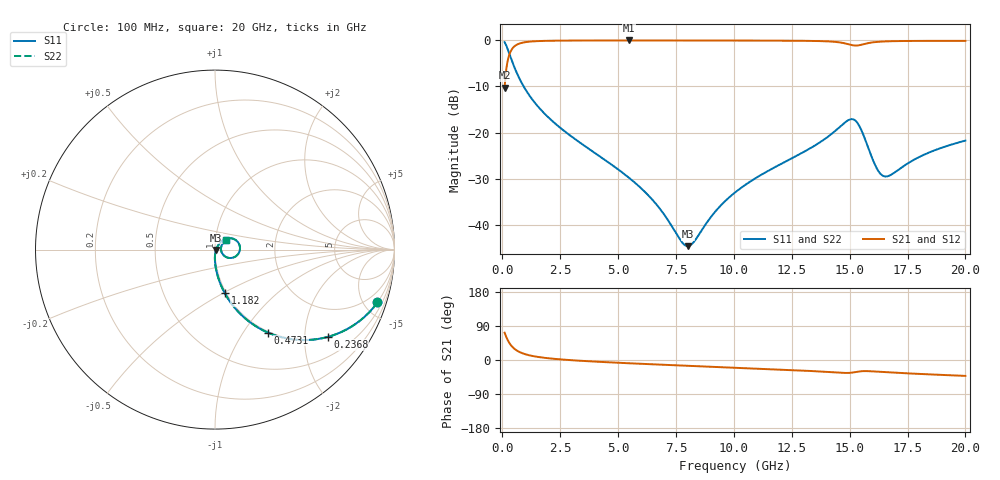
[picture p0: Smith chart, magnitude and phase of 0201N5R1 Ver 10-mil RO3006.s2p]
# GHz S MA R 50
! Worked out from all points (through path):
!   1601 points, 100 MHz to 20 GHz, reference 50 ohm
!   highest |S21| = -0.05 dB at 5.485 GHz (marker M1); lowest = -10.3 dB at 100 MHz (marker M2)
!   group delay of S21, straight-line fit = 7.98 ps
!   lowest |S11| = -44.6 dB at 8.01 GHz (marker M3), VSWR 1.01, Z = 50.6 - j0.179 ohm
!   |S11| at or under -10 dB: 921.4 MHz to end of sweep
!   |S22| runs from -44.6 to -0.4 dB; largest |S21 - S12| = 0
!   S11 on the Smith chart (normalised r, x): 100 MHz: 0.98, -6.16; 236.8 MHz: 0.98, -2.60; 473.1 MHz: 0.98, -1.30; 1.182 GHz: 0.98, -0.51; 20 GHz: 1.13, +0.12
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0.1  0.9519 -18.0  0.3057 72.0  0.3057 72.0  0.9519 -18.0
0.2368125  0.7952 -37.7  0.6052 52.2  0.6052 52.2  0.7952 -37.7
0.473125  0.5479 -57.5  0.835 32.3  0.835 32.3  0.5479 -57.5
0.74675  0.3817 -68.7  0.9225 21.0  0.9225 21.0  0.3817 -68.7
1.182063  0.2496 -77.3  0.9661 12.2  0.9661 12.2  0.2496 -77.3
2.077562  0.1392 -84.8  0.9874 4.0  0.9874 4.0  0.1392 -84.8
3.420812  0.07566 -89.4  0.9934 -2.2  0.9934 -2.2  0.07566 -89.4
5.485437  0.03214 -90.2  0.9946 -8.7  0.9946 -8.7  0.03214 -90.2
6.741625  0.01566 -82.3  0.9944 -12.0  0.9944 -12.0  0.01566 -82.3
7.724188  0.00665 -45.0  0.9941 -14.5  0.9941 -14.5  0.00665 -45.0
8.01025  0.005871 -17.6  0.9939 -15.3  0.9939 -15.3  0.005871 -17.6
8.283875  0.006576 8.3  0.9938 -15.9  0.9938 -15.9  0.006576 8.3
9.291313  0.01481 45.5  0.9932 -18.4  0.9932 -18.4  0.01481 45.5
10.05  0.02241 51.6  0.9926 -20.3  0.9926 -20.3  0.02241 51.6
13.37081  0.06918 49.1  0.9833 -29.2  0.9833 -29.2  0.06918 49.1
14.61456  0.1174 31.2  0.9441 -33.7  0.9441 -33.7  0.1174 31.2
15.16181  0.1387 -0.2  0.88 -32.9  0.88 -32.9  0.1387 -0.2
15.47275  0.1108 -23.6  0.8894 -29.8  0.8894 -29.8  0.1108 -23.6
16.23144  0.03859 -19.7  0.9617 -31.0  0.9617 -31.0  0.03859 -19.7
16.69162  0.03392 10.6  0.9746 -32.7  0.9746 -32.7  0.03392 10.6
18.19656  0.05726 38.7  0.9842 -37.3  0.9842 -37.3  0.05726 38.7
20  0.0818 39.8  0.9845 -41.9  0.9845 -41.9  0.0818 39.8
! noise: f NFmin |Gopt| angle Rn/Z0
0.1  0.0009112  0.9526  0.4028  0.004326
2.301  0.005231  0.822  4.547  0.006155
4.515  0.008695  0.7935  8.714  0.008647
6.729  0.01181  0.7764  12.88  0.01067
8.943  0.01488  0.7664  17.01  0.01267
11.14  0.01846  0.7666  21.09  0.01556
13.36  0.02694  0.8054  25.17  0.02742
15.57  0.07942  0.9188  29.33  0.2022
17.79  0.03213  0.788  33.26  0.02868
20  0.02999  0.752  37.11  0.02197
